(* Logix 5000 AddOnInstructionDefinition export AMCI_MA_Preset_Encoder; software revision 20.05 *)

TYPE AMCI_Motion_Axis_Output_Data :
STRUCT
   Control_Word_0 : INT;
   Control_Word_1 : INT;
   Position_or_Distance : DINT;
   Programmed_Speed : DINT;
   Acceleration : INT;
   Deceleration : INT;
   Output_Word_8 : INT;
   Output_Word_9 : INT;
END_STRUCT
END_TYPE

TYPE AMCI_Motion_Axis_Input_Data :
STRUCT
   Moving_CW : BOOL;
   Moving_CCW : BOOL;
   In_Hold_State : BOOL;
   Stopped : BOOL;
   At_Home : BOOL;
   Accelerating : BOOL;
   Decelerating : BOOL;
   Move_Complete : BOOL;
   Status_Word_0_Bit_8 : BOOL;
   Status_Word_0_Bit_9 : BOOL;
   Position_Invalid : BOOL;
   Input_Error : BOOL;
   Command_Error : BOOL;
   Configuration_Error : BOOL;
   Module_OK : BOOL;
   Mode_Flag : BOOL;
   IN1_Active : BOOL;
   IN2_Active : BOOL;
   IN3_Active : BOOL;
   IN4_Active : BOOL;
   Status_Word_1_Bit_4 : BOOL;
   Status_Word_1_Bit_5 : BOOL;
   Connection_Was_Lost : BOOL;
   Driver_Fault : BOOL;
   Status_Word_1_Bit_8 : BOOL;
   Invalid_Jog_Change : BOOL;
   Status_Word_1_Bit_10 : BOOL;
   Heartbeat_Bit : BOOL;
   Status_Word_1_Bit_12 : BOOL;
   Status_Word_1_Bit_13 : BOOL;
   Stall_Detected : BOOL;
   Drive_Is_Enabled : BOOL;
   Motor_Position : DINT;
   Encoder_Position : DINT;
   Trapped_Encoder_Position : DINT;
   Input_Word_8 : INT;
   Input_Word_9 : INT;
END_STRUCT
END_TYPE

ADD_ON_INSTRUCTION AMCI_MA_Preset_Encoder   (* revision 2.1, vendor AMCI, ExecuteEnableInFalse *)
// AMCI Preset Encoder Position.  Will not work on SVXXXE2
// Revision note:
// 3/6/23: Added Save in Flash bit
// 11/17/23 V2.1 Reset output word 0 to 0 when the rung goes false.
// Help:
// MOTION_AXIS_PRESET_ENCODER: Preset Encoder Position to a value.  This AOI will only work on AMCI SD and SMD devices that have an encoder.   This AOI WILL NOT WORK  with SVXXXE2 units
// Note: This instruction will maintain the motion device’s current enabled state.  That is, if the device is enabled,
//            it will remain enabled.  If it is disabled, it will remain disabled.
// AXIS INPUT DATA:  Input data from AMCI motion device.   Uses the AMCI_Motion_Axis_Input_Data User Defined Data Type.
// AXIS OUTPUT DATA; Output data from the AOI to the AMCI motion device.   Uses the AMCI_Motion_Axis_Output_Data User Defined Data Type.
// POSITION: Position to which the Encoder Position is to be set.
// SAVE_IN_FLASH_0_NO_1_YES:  Saves the offset encoder value in the flash memory.    Only used on the SMDXXE2 units with Absolute Encoders.  Must be zero on all other units.
// EN (Enable) Set when rung is true, Reset when rung is false
// DN (Done) Set when command is sent to the motion device.  Reset when the rung is false.
// ER (Error) Set when a command or input error failed to clear.  Reset when the rung is false.
VAR_IN_OUT
   Axis_Input_Data : AMCI_Motion_Axis_Input_Data; {required}
        [0].6   // set when decelerating
   Axis_Output_Data : AMCI_Motion_Axis_Output_Data; {required}
END_VAR
VAR_INPUT
   Position : DINT; {required}
   save_in_flash_0_no_1_yes : BOOL; {required}
END_VAR
VAR_OUTPUT
   EN : BOOL; {visible}   // set when rung with AOI is true
   DN : BOOL; {access Read Only, visible}   // set when preset motor position command sent to motion axis
   ER : BOOL; {access Read Only, visible}   // set when input, command, or configuraiton error
END_VAR
VAR
   command_data_block : INT[10];
        [0]   // Command Bits MSW
        [1]   // Command Bits LSW
        [2]   // Upper Target Position
        [3]   // Lower Target Position
        [4]   // Upper Programmed Speed
        [5]   // Lower Programmed Speed
END_VAR

ROUTINE EnableInFalse   (* ladder *)
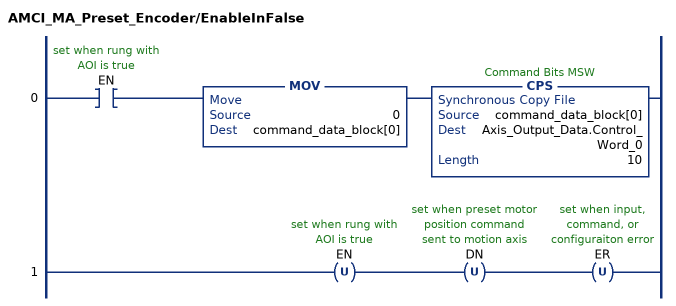
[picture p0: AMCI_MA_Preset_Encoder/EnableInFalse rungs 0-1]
   0: XIC(EN)MOV(0,command_data_block[0])CPS(command_data_block[0],Axis_Output_Data.Control_Word_0,10);
   1: OTU(EN)OTU(DN)OTU(ER);
END_ROUTINE

ROUTINE Logic   (* ladder *)
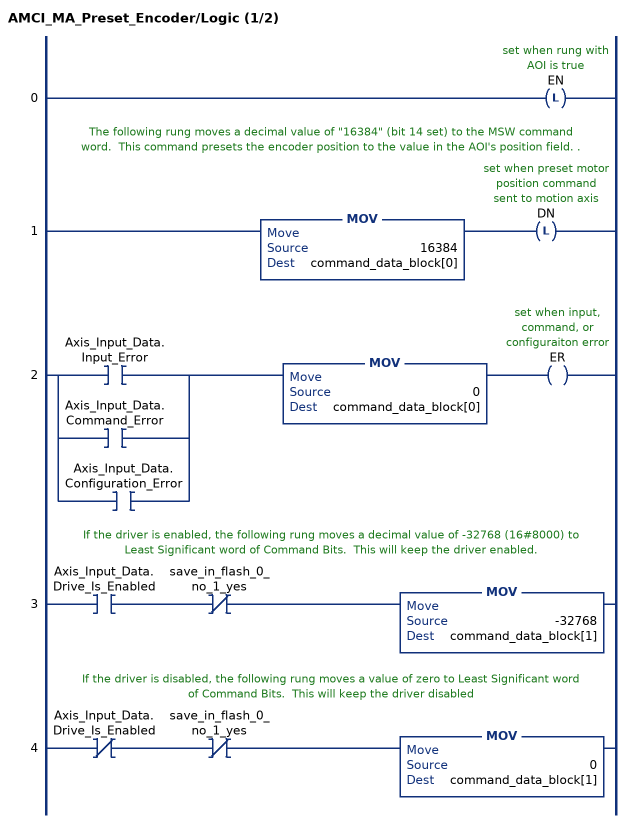
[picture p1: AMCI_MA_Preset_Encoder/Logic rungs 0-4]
   0: OTL(EN);
   // The following rung moves a decimal value of "16384" (bit 14 set) to the MSW command word.  This command presets the encoder position to the value in the AOI's position field. .
   1: MOV(16384,command_data_block[0])OTL(DN);
   2: [XIC(Axis_Input_Data.Input_Error) ,XIC(Axis_Input_Data.Command_Error) ,XIC(Axis_Input_Data.Configuration_Error) ]MOV(0,command_data_block[0])OTE(ER);
   // If the driver is enabled, the following rung moves a decimal value of -32768 (16#8000) to Least Significant word of Command Bits.  This will keep the driver enabled.
   3: XIC(Axis_Input_Data.Drive_Is_Enabled)XIO(save_in_flash_0_no_1_yes)MOV(-32768,command_data_block[1]);
   // If the driver is disabled, the following rung moves a value of zero to Least Significant word of Command Bits.  This will keep the driver disabled
   4: XIO(Axis_Input_Data.Drive_Is_Enabled)XIO(save_in_flash_0_no_1_yes)MOV(0,command_data_block[1]);
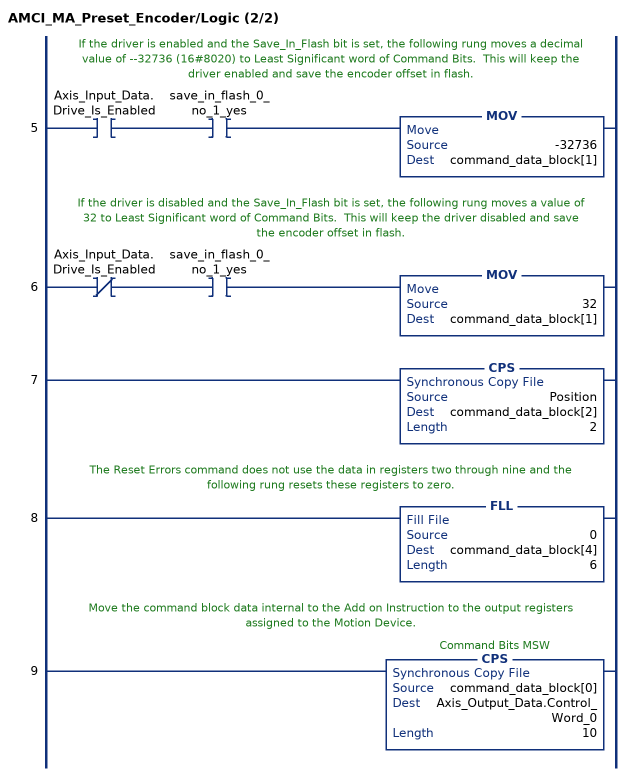
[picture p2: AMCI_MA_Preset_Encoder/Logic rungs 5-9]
   // If the driver is enabled and the Save_In_Flash bit is set, the following rung moves a decimal value of --32736 (16#8020) to Least Significant word of Command Bits.  This will keep the driver enabled and save the encoder offset in flash.
   5: XIC(Axis_Input_Data.Drive_Is_Enabled)XIC(save_in_flash_0_no_1_yes)MOV(-32736,command_data_block[1]);
   // If the driver is disabled and the Save_In_Flash bit is set, the following rung moves a value of 32 to Least Significant word of Command Bits.  This will keep the driver disabled and save the encoder offset in flash.
   6: XIO(Axis_Input_Data.Drive_Is_Enabled)XIC(save_in_flash_0_no_1_yes)MOV(32,command_data_block[1]);
   7: CPS(Position,command_data_block[2],2);
   // The Reset Errors command does not use the data in registers two through nine and the following rung resets these registers to zero.
   8: FLL(0,command_data_block[4],6);
   // Move the command block data internal to the Add on Instruction to the output registers assigned to the Motion Device.
   9: CPS(command_data_block[0],Axis_Output_Data.Control_Word_0,10);
END_ROUTINE
END_ADD_ON_INSTRUCTION
